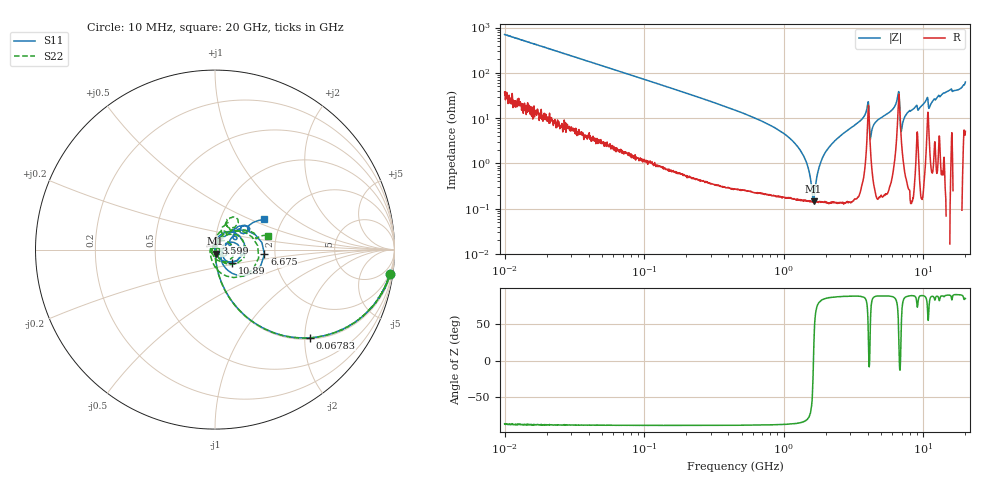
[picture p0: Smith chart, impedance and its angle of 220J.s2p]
!Keysight Technologies,P5008B,MY61100088,A.16.20.02
!Date: Tuesday, November 07, 2023 15:46:02
!Correction: S11(C  2-Port  )
!S21(C  2-Port  )
!S12(C  2-Port  )
!S22(C  2-Port  )
!S2P File: Measurements: S11, S21, S12, S22:Log Frequency Sweep
# Hz S  dB  R 50
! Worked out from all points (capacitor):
!   1601 points, 10 MHz to 20 GHz, reference 50 ohm
!   read as one part in series: C = 22.6 pF near 10.39 MHz
!   lowest |Z| = 147 mohm at 1.636 GHz (marker M1)
!   series resonance near 1.631 GHz, so ESL is about 420 pH
!   S11 on the Smith chart (normalised r, x): 10 MHz: 2, -14; 67.83 MHz: 1.04, -2.11; 3.599 GHz: 1.00, +0.08; 6.675 GHz: 1.76, -0.10; 10.89 GHz: 1.19, -0.17; 20 GHz: 1.62, +0.61
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1e7  -0.15 -8.0  -17.09 78.9  -17.09 79.0  -0.15 -8.0
3.555162e7  -1.05 -26.3  -7.08 62.3  -7.08 62.4  -1.04 -26.4
6.783392e7  -2.85 -42.9  -3.35 45.9  -3.35 45.9  -2.85 -43.0
1.263918e8  -6.17 -59.8  -1.28 29.2  -1.28 29.2  -6.17 -60.0
4.472136e8  -16.20 -80.7  -0.13 8.1  -0.13 8.1  -16.20 -81.0
1.589917e9  -32.07 -82.6  -0.01 -1.2  -0.02 -1.2  -32.03 -92.8
1.635887e9  -32.70 -81.6  -0.01 -1.4  -0.02 -1.3  -32.70 -93.7
2.134466e9  -41.26 -70.2  -0.01 -3.2  -0.01 -3.2  -41.18 -95.6
2.461408e9  -57.26 -8.5  -0.01 -4.3  -0.01 -4.3  -53.61 -35.4
2.87917e9  -39.31 93.7  -0.01 -5.7  -0.01 -5.7  -39.42 54.9
3.599441e9  -28.46 87.5  -0.03 -8.5  -0.03 -8.5  -28.51 64.7
4.034136e9  -15.54 11.5  -1.55 -10.3  -1.55 -10.3  -15.17 2.7
4.478574e9  -48.83 105.9  -0.02 -8.7  -0.02 -8.7  -41.12 12.3
5.652411e9  -30.13 65.8  -0.01 -13.3  -0.01 -13.3  -29.68 71.9
6.674885e9  -11.16 -5.3  -2.56 -15.8  -2.56 -15.7  -12.12 -10.9
7.340179e9  -26.41 -46.5  -0.03 -13.7  -0.04 -13.6  -29.73 -141.4
8.5048e9  -32.07 -19.1  0.01 -18.8  0.01 -18.8  -36.71 162.6
9.807503e9  -31.06 0.8  0.02 -22.2  0.01 -22.2  -35.11 128.4
1.088799e10  -18.55 -37.7  -0.72 -20.9  -0.72 -20.9  -22.11 -62.2
1.141771e10  -27.27 -2.8  -0.03 -24.6  -0.03 -24.6  -33.54 119.8
1.393898e10  -15.14 39.9  -0.15 -32.6  -0.15 -32.6  -15.54 64.8
2e10  -9.81 31.5  -1.00 -57.8  -1.00 -57.7  -10.27 14.5
